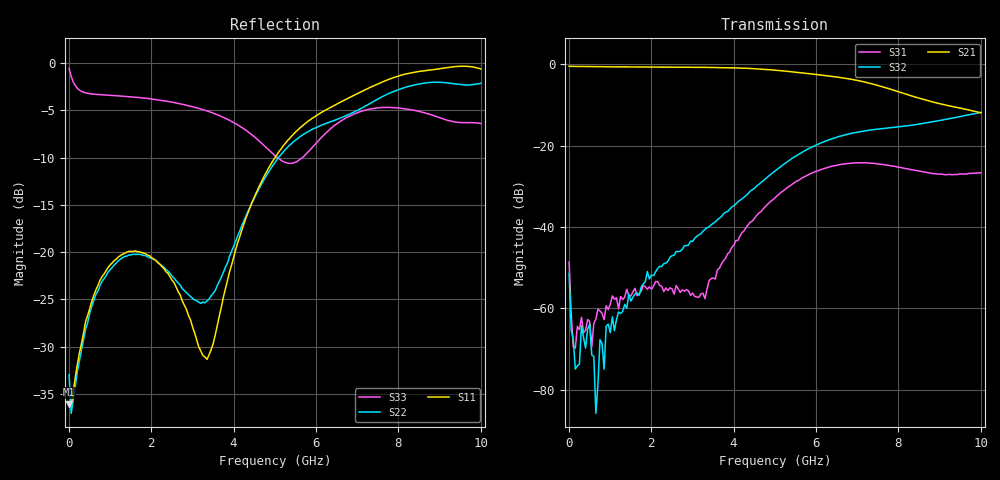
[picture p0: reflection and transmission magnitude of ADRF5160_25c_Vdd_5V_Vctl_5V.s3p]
! Device:  ADRF5160
! Description: Silicon SPDT Switch
! Frequency:  0.7 -  4 GHz
! Ports:
!	RFc	= Port 1
!	RF1	= Port 2
!  RF2  = Port 3
! Vdd:  5 Volt
! Control:  5 Volt
! Data:  Data was collected using a calibrated 4 port network analyzer and de-embedded using Agilent's AFR De-Embedding.
! Note:  Analog Devices supplies this data as a sample of measured data
!  for this product.  Your particular data for this product may vary.
!  Data was taken at 25 degrees C.
!S3P File: Measurements: <S11,S12,S13>,
!<S21,S22,S23>,
!<S31,S32,S33>:
# Hz S  dB  R 50
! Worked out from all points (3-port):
!   201 points, 10 MHz to 10 GHz, reference 50 ohm
!   strongest paths, dB at 10 MHz, 2.507 GHz, 5.005 GHz, 7.503 GHz, 10 GHz:
!     S21: -0.5, -0.7, -1.4, -5.2, -11.9
!     S32: -51.4, -47.1, -26.2, -15.9, -11.8
!     S31: -48.6, -55.3, -32.9, -24.5, -26.7
!   lowest |S11| = -36.1 dB at 10 MHz (marker M1), VSWR 1.03, Z = 51.6 + j0.00853 ohm
!   |S11| at or under -10 dB: start of sweep to 5.009 GHz
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1e7  -36.11 0.3  -0.50 -0.5  -51.87 59.0
     -0.45 -0.4  -32.96 -12.6  -47.66 19.7
     -48.65 -81.6  -51.44 -39.9  -0.59 -9.0
1.099e8  -34.79 -45.8  -0.50 -3.0  -69.59 162.7
         -0.51 -3.0  -35.58 -47.7  -73.20 12.7
         -69.47 79.3  -67.60 -45.0  -2.01 -73.8
1.5985e8  -33.23 -55.4  -0.51 -4.3  -69.52 30.2
          -0.52 -4.3  -34.24 -57.3  -72.85 -6.6
          -69.86 85.3  -74.97 55.8  -2.40 -94.8
5.095e8  -25.98 -84.7  -0.55 -13.2  -63.39 74.6
         -0.55 -13.3  -26.47 -90.8  -65.56 -37.3
         -63.28 170.4  -63.94 -32.1  -3.24 -154.0
6.5935e8  -24.00 -92.7  -0.56 -17.1  -64.31 79.6
          -0.56 -17.1  -24.46 -99.7  -69.19 -145.7
          -62.64 65.3  -85.85 34.8  -3.32 -164.0
1.05895e9  -21.12 -104.4  -0.61 -27.2  -59.65 70.0
           -0.61 -27.2  -21.59 -114.5  -61.97 -133.4
           -56.98 82.7  -62.12 -125.5  -3.44 179.4
3.35665e9  -31.34 137.5  -0.75 -87.2  -55.68 133.2
           -0.75 -87.2  -25.16 -132.6  -40.04 175.5
           -55.26 132.0  -40.22 175.4  -5.08 123.9
5.005e9  -10.02 16.2  -1.43 -136.1  -32.83 119.0
         -1.43 -136.1  -10.52 -119.3  -26.22 135.5
         -32.86 118.7  -26.24 135.2  -9.81 95.6
7.5025e9  -2.21 -48.1  -5.20 146.4  -24.49 -15.8
          -5.20 146.5  -3.81 154.2  -15.91 19.1
          -24.49 -15.8  -15.92 19.2  -4.75 77.7
1e10  -0.64 -79.3  -11.93 95.8  -26.70 -76.9
      -11.93 95.9  -2.14 90.8  -11.80 -62.8
      -26.67 -76.4  -11.81 -62.6  -6.41 1.5
